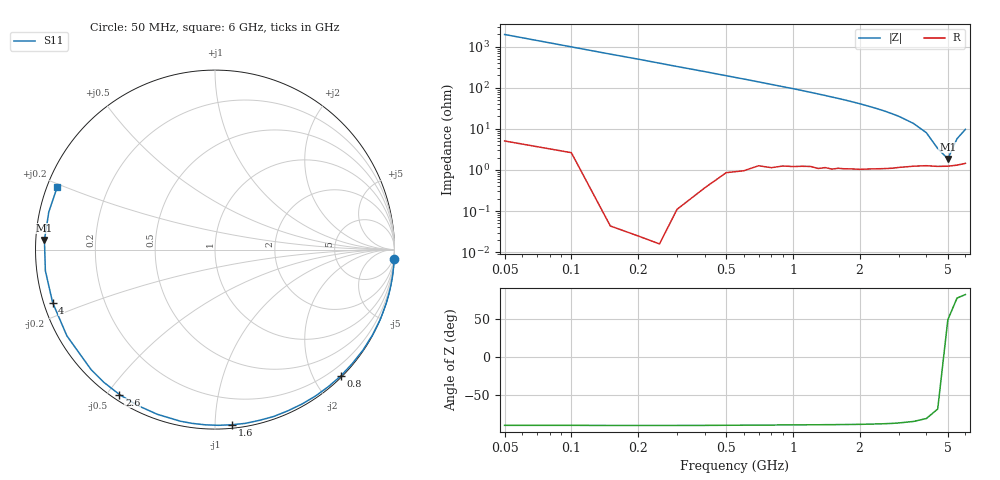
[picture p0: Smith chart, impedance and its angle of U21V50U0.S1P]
! SIEMENS Discrete & RF Semiconductors
! BBY52-02W
! Si Tuning Diode in SCD-80
! VR = 1.5 V
! S-Parameters:  September  1997
# GHz  S  MA  R  50
!  f  S11
! GHz  MAG  ANG
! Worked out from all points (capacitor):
!   34 points, 50 MHz to 6 GHz, reference 50 ohm
!   read as one part to ground: C = 1.61 pF near 50 MHz
!   lowest |Z| = 1.86 ohm at 5 GHz (marker M1)
!   series resonance near 4.845 GHz, so ESL is about 670 pH
!   S11 on the Smith chart (normalised r, x): 50 MHz: 0, -40; 800 MHz: 0.02, -2.41; 1.6 GHz: 0.02, -1.10; 2.6 GHz: 0.02, -0.54; 4 GHz: 0.03, -0.16; 6 GHz: 0.03, +0.19
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0.05  0.9999 -2.9
0.2  1 -11.5
0.3  0.9999 -17.3
0.4  0.9994 -22.9
0.5  0.9979 -28.6
0.6  0.9967 -34.1
0.8  0.9933 -45.1
0.9  0.991 -50.4
1  0.9895 -55.5
1.1  0.9876 -60.6
1.2  0.9858 -65.7
1.3  0.9856 -70.6
1.4  0.983 -75.4
1.5  0.9828 -80.1
1.6  0.9803 -84.5
1.8  0.9777 -93.2
2  0.9755 -101.4
2.2  0.9722 -109.3
2.4  0.9695 -116.5
2.6  0.967 -123.4
2.8  0.9644 -129.9
3  0.9612 -135.9
3.5  0.955 -149.8
4  0.9516 -161.9
4.5  0.9524 -172.9
5  0.9518 176.8
5.5  0.9495 167.2
6  0.9457 158.2
